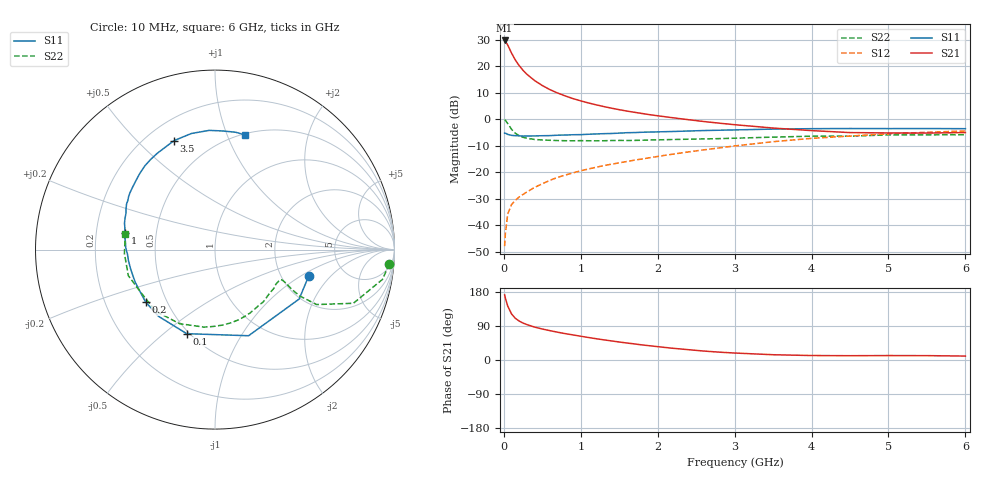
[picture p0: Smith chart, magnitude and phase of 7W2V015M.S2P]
! Infineon Technologies  Discrete & RF Semiconductors
! BFS17W
! Si NPN RF Bipolar Junction Transistor in SOT323
! VCE = 2 V  IC = 15 mA
! Common Emitter S-Parameters:  August  1999
# GHz  S  MA  R  50
!  f  S11  S21  S12  S22
! GHz  MAG  ANG  MAG  ANG  MAG  ANG  MAG  ANG
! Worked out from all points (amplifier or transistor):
!   36 points, 10 MHz to 6 GHz, reference 50 ohm
!   highest |S21| = 29.7 dB at 10 MHz (marker M1)
!   |S21| within 3 dB of that: start of sweep to 71.29 MHz
!   unconditionally stable (mu >= 1): 292.6 MHz to 2.805 GHz; 4.093 GHz to end of sweep
!   at 250 MHz: K = 0.93, MSG = 23.4 dB, |S12| = -28.4 dB
!   at 1.4 GHz: K = 1.23, MAG = 7.7 dB, |S12| = -17.0 dB
!   at 6 GHz: K = 1.09, MAG = -2.1 dB, |S12| = -4.5 dB
!   S11 on the Smith chart (normalised r, x): 10 MHz: 2.84, -1.17; 100 MHz: 0.48, -0.60; 200 MHz: 0.38, -0.29; 1 GHz: 0.33, +0.08; 3.5 GHz: 0.31, +0.65; 6 GHz: 0.51, +1.16
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0.01  0.5427 -15.5  30.54 171.9  0.004 81.7  0.9747 -4.7
0.02  0.5438 -30.4  29.64 163.3  0.0069 81.1  0.9476 -10.1
0.05  0.5151 -68.7  25.11 142.5  0.0161 66.1  0.827 -21.2
0.1  0.4942 -108.6  17.66 121.6  0.0244 56.3  0.6438 -28.4
0.15  0.4871 -130.3  13.02 109.9  0.0294 53.8  0.5396 -28.7
0.2  0.4844 -142.9  10.2 102.7  0.034 55.7  0.4864 -27.5
0.25  0.4786 -151.7  8.327 97.4  0.038 57.5  0.4533 -26.1
0.3  0.4803 -158.0  7.023 93.4  0.0421 58.8  0.4356 -25.2
0.4  0.4822 -166.8  5.341 86.8  0.0515 62.1  0.4129 -24.4
0.5  0.4861 -172.7  4.306 81.8  0.0602 63.7  0.4044 -24.5
0.6  0.4884 -177.1  3.595 77.4  0.0701 64.8  0.3983 -25.5
0.7  0.4974 178.8  3.107 73.3  0.0796 65.7  0.3941 -27.1
0.8  0.5008 175.1  2.735 69.5  0.0881 66.3  0.3912 -29.0
1  0.5099 169.3  2.21 62.7  0.1059 67.1  0.3927 -33.2
1.1  0.5182 165.9  2.019 59.3  0.1147 66.9  0.3906 -36.2
1.6  0.5542 152.8  1.419 44.8  0.1586 67.3  0.3945 -50.9
2.2  0.5844 139.0  1.059 30.9  0.2185 66.5  0.4124 -70.8
2.8  0.6174 125.4  0.839 20.7  0.2865 63.1  0.4286 -91.5
3.5  0.6485 110.7  0.679 13.9  0.3749 56.7  0.4575 -115.5
4.5  0.665 92.8  0.557 11.3  0.4788 43.8  0.4769 -149.6
5.5  0.6639 80.0  0.545 11.5  0.5638 31.6  0.5052 -177.5
6  0.6601 75.3  0.558 10.4  0.5982 25.8  0.507 170.3
